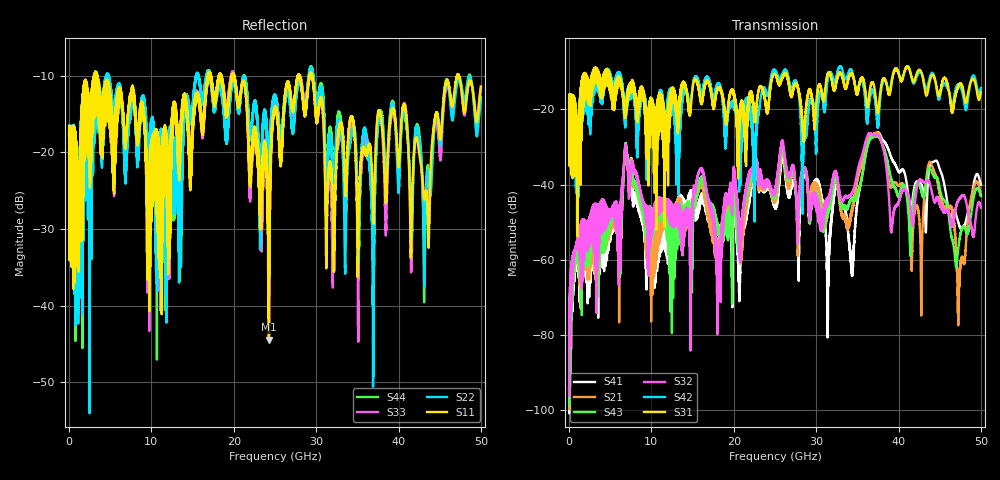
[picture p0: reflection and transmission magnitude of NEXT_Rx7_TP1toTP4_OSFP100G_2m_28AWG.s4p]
! Touchstone data
! Created: 27-Feb-2019 by IdEM 12 (12.1.0)
! COMMENTS
!  Created Wed Feb 27 12:03:36 2019
!  64 Port Network Data from SP1.SP block
!  freq  magS1_1  angS1_1  magS1_2  angS1_2  magS1_3  angS1_3  magS1_4  angS1_4
!  magS1_5  angS1_5  magS1_6  angS1_6  magS1_7  angS1_7  magS1_8  angS1_8
!  magS1_9  angS1_9  magS1_10  angS1_10  magS1_11  angS1_11  magS1_12  angS1_12
!  magS1_13  angS1_13  magS1_14  angS1_14  magS1_15  angS1_15  magS1_16  angS1_16
!  magS1_17  angS1_17  magS1_18  angS1_18  magS1_19  angS1_19  magS1_20  angS1_20
!  magS1_21  angS1_21  magS1_22  angS1_22  magS1_23  angS1_23  magS1_24  angS1_24
!  magS1_25  angS1_25  magS1_26  angS1_26  magS1_27  angS1_27  magS1_28  angS1_28
!  magS1_29  angS1_29  magS1_30  angS1_30  magS1_31  angS1_31  magS1_32  angS1_32
!  magS1_33  angS1_33  magS1_34  angS1_34  magS1_35  angS1_35  magS1_36  angS1_36
!  magS1_37  angS1_37  magS1_38  angS1_38  magS1_39  angS1_39  magS1_40  angS1_40
!  magS1_41  angS1_41  magS1_42  angS1_42  magS1_43  angS1_43  magS1_44  angS1_44
!  magS1_45  angS1_45  magS1_46  angS1_46  magS1_47  angS1_47  magS1_48  angS1_48
!  magS1_49  angS1_49  magS1_50  angS1_50  magS1_51  angS1_51  magS1_52  angS1_52
!  magS1_53  angS1_53  magS1_54  angS1_54  magS1_55  angS1_55  magS1_56  angS1_56
!  magS1_57  angS1_57  magS1_58  angS1_58  magS1_59  angS1_59  magS1_60  angS1_60
!  magS1_61  angS1_61  magS1_62  angS1_62  magS1_63  angS1_63  magS1_64  angS1_64
!  magS2_1  angS2_1  magS2_2  angS2_2  magS2_3  angS2_3  magS2_4  angS2_4
!  magS2_5  angS2_5  magS2_6  angS2_6  magS2_7  angS2_7  magS2_8  angS2_8
!  magS2_9  angS2_9  magS2_10  angS2_10  magS2_11  angS2_11  magS2_12  angS2_12
!  magS2_13  angS2_13  magS2_14  angS2_14  magS2_15  angS2_15  magS2_16  angS2_16
!  magS2_17  angS2_17  magS2_18  angS2_18  magS2_19  angS2_19  magS2_20  angS2_20
!  magS2_21  angS2_21  magS2_22  angS2_22  magS2_23  angS2_23  magS2_24  angS2_24
!  magS2_25  angS2_25  magS2_26  angS2_26  magS2_27  angS2_27  magS2_28  angS2_28
!  magS2_29  angS2_29  magS2_30  angS2_30  magS2_31  angS2_31  magS2_32  angS2_32
!  magS2_33  angS2_33  magS2_34  angS2_34  magS2_35  angS2_35  magS2_36  angS2_36
!  magS2_37  angS2_37  magS2_38  angS2_38  magS2_39  angS2_39  magS2_40  angS2_40
!  magS2_41  angS2_41  magS2_42  angS2_42  magS2_43  angS2_43  magS2_44  angS2_44
!  magS2_45  angS2_45  magS2_46  angS2_46  magS2_47  angS2_47  magS2_48  angS2_48
!  magS2_49  angS2_49  magS2_50  angS2_50  magS2_51  angS2_51  magS2_52  angS2_52
!  magS2_53  angS2_53  magS2_54  angS2_54  magS2_55  angS2_55  magS2_56  angS2_56
!  magS2_57  angS2_57  magS2_58  angS2_58  magS2_59  angS2_59  magS2_60  angS2_60
!  magS2_61  angS2_61  magS2_62  angS2_62  magS2_63  angS2_63  magS2_64  angS2_64
!  magS3_1  angS3_1  magS3_2  angS3_2  magS3_3  angS3_3  magS3_4  angS3_4
!  magS3_5  angS3_5  magS3_6  angS3_6  magS3_7  angS3_7  magS3_8  angS3_8
!  magS3_9  angS3_9  magS3_10  angS3_10  magS3_11  angS3_11  magS3_12  angS3_12
!  magS3_13  angS3_13  magS3_14  angS3_14  magS3_15  angS3_15  magS3_16  angS3_16
!  magS3_17  angS3_17  magS3_18  angS3_18  magS3_19  angS3_19  magS3_20  angS3_20
!  magS3_21  angS3_21  magS3_22  angS3_22  magS3_23  angS3_23  magS3_24  angS3_24
!  magS3_25  angS3_25  magS3_26  angS3_26  magS3_27  angS3_27  magS3_28  angS3_28
!  magS3_29  angS3_29  magS3_30  angS3_30  magS3_31  angS3_31  magS3_32  angS3_32
!  magS3_33  angS3_33  magS3_34  angS3_34  magS3_35  angS3_35  magS3_36  angS3_36
!  magS3_37  angS3_37  magS3_38  angS3_38  magS3_39  angS3_39  magS3_40  angS3_40
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# Hz S MA R 50
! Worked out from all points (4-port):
!   5000 points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, 10 MHz to 50 GHz, reference 50 ohm
!   strongest paths, dB at 10 MHz, 12.51 GHz, 25.01 GHz, 37.51 GHz, 50 GHz:
!     S31: -18.0, -15.9, -10.7, -20.7, -15.4
!     S42: -18.0, -16.4, -9.6, -24.1, -14.3
!     S32: -92.0, -45.2, -41.6, -26.8, -46.1
!     S43: -94.1, -49.1, -43.6, -27.2, -42.8
!     S21: -93.7, -46.1, -44.4, -26.2, -43.0
!     S41: -94.4, -48.6, -46.2, -26.1, -40.0
!   lowest |S11| = -44.4 dB at 24.26 GHz (marker M1), VSWR 1.01, Z = 49.6 - j0.401 ohm
!   |S11| at or under -10 dB: 3.451 GHz to 16.86 GHz (13.4 GHz wide, 132 % of centre); 20.09 GHz to 27.79 GHz (7.695 GHz wide, 32.1 % of centre); 29.5 GHz to 47.1 GHz (17.61 GHz wide, 46 % of centre)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
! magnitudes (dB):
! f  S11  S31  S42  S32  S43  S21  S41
! 10 MHz  -17.7  -18.0  -18.0  -92.0  -94.1  -93.7  -94.4
! 6.89 GHz  -18.1  -21.6  -20.6  -29.5  -29.1  -29.3  -29.0
! 18.15 GHz  -10.4  -14.0  -13.1  -59.5  -51.4  -54.6  -51.8
! 24.26 GHz  -44.4  -18.3  -15.0  -39.3  -39.8  -39.2  -40.5
! 37.46 GHz  -15.2  -20.9  -24.1  -26.8  -27.2  -26.2  -26.1
! 47.32 GHz  -10.0  -13.5  -13.5  -44.1  -55.8  -68.4  -50.5
! 50 GHz  -11.4  -15.4  -14.3  -46.1  -42.8  -43.0  -40.0
